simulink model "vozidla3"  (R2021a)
settings: Solver=VariableStepAuto  StartTime=0.0  StopTime=10  RelTol=1e-5
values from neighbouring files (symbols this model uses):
  Az = A-B*K    [appDekompLQR.m]    (also in appLQR.m; appSYM.m = A+B*K; appSZV.m = A+B*K; central_LQR.m)
  C = eye(pocet_stavu)    [appDekompLQR.m]    (also in appLQR.m; appSYM.m; appSZV.m; central_LQR.m)
  conds = [0 , 4 , 0 , 2 , 0, 1, 0, -1, 0]    [central_LQR.m]    (also in central_SYM.m = [0 , 4 , 0 , 3 , 0, 2, 0, -1, 0]; distri_STRUKTURAL.m = [0 , 4 , 0 , 3 , 0, 2, 0, -1, 0]; distri_SZV.m = [0 , 4 , 0 , 3 , 0, 2, 0, -1, 0]; porovnani_rizeni.m)
  conds0 = zeros(1,2*N-1)    [central_LQR.m]    (also in central_SYM.m; distri_STRUKTURAL.m = zeros(1,pocet_stavu); distri_SZV.m; porovnani_rizeni.m)
  D = zeros(pocet_stavu,N)    [appDekompLQR.m]    (also in appLQR.m; appSYM.m; appSZV.m; central_LQR.m)
  porucha = B    [appDekompLQR.m]    (also in appLQR.m; appSYM.m; appSZV.m; central_LQR.m)
libraries: simulink x1

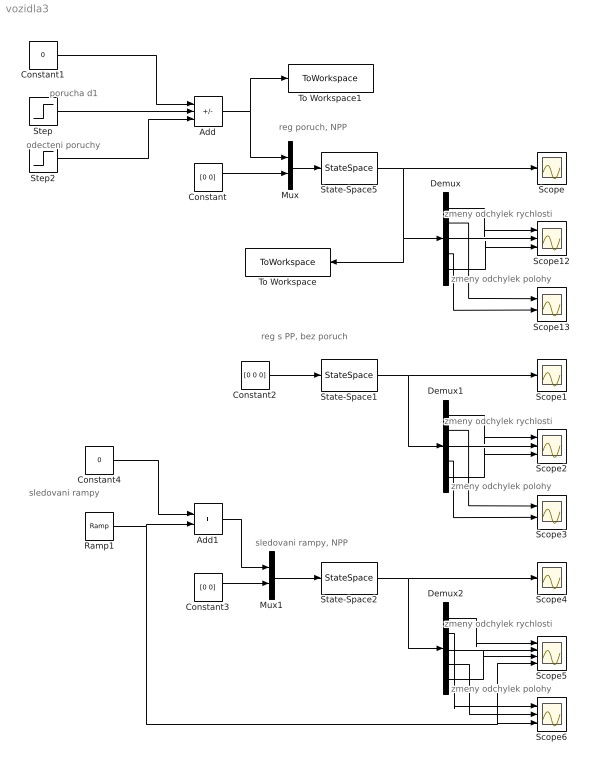
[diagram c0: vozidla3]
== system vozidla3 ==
  note: reg poruch, NPP
  note: reg s PP, bez poruch
  note: odecteni poruchy
  note: porucha d1
  note: zmeny odchylek polohy
  note: zmeny odchylek rychlosti
  note: zmeny odchylek polohy
  note: zmeny odchylek rychlosti
  note: sledovani rampy, NPP
  note: zmeny odchylek polohy
  note: zmeny odchylek rychlosti
  note: sledovani rampy
  Add : Sum  Inputs=++-
  Add1 : Sum
  Constant : Constant  Value=[0 0]
  Constant1 : Constant  Value=0
  Constant2 : Constant  Value=[0 0 0]
  Constant3 : Constant  Value=[0 0]
  Constant4 : Constant  Value=0
  Demux : Demux  Outputs=5
  Demux1 : Demux  Outputs=5
  Demux2 : Demux  Outputs=5
  Mux : Mux  Inputs=2
  Mux1 : Mux  Inputs=2
  Ramp1 : simulink/Sources/Ramp  slope=1  start=5  InitialOutput=0
  Scope : Scope
  Scope1 : Scope
  Scope12 : Scope  NumInputPorts=3
  Scope13 : Scope  NumInputPorts=2
  Scope2 : Scope  NumInputPorts=3
  Scope3 : Scope  NumInputPorts=2
  Scope4 : Scope
  Scope5 : Scope  NumInputPorts=4
  Scope6 : Scope  NumInputPorts=3
  State-Space1 : StateSpace  A=Az  B=porucha  C=C  D=D  InitialCondition=conds
  State-Space2 : StateSpace  A=Az  B=porucha  C=C  D=D  InitialCondition=conds0
  State-Space5 : StateSpace  A=Az  B=porucha  C=C  D=D  InitialCondition=conds0
  Step : Step  Time=5  After=2  SampleTime=0
  Step2 : Step  Time=6  After=2  SampleTime=0
  To Workspace : ToWorkspace  VariableName=stavy  SaveFormat=Structure  SampleTime=-1
  To Workspace1 : ToWorkspace  VariableName=vstup  SaveFormat=Structure  SampleTime=-1
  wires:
  State-Space5/1 -> Scope/1, To Workspace/1, Demux/1
  Demux/1 -> Scope12/1
  Demux/3 -> Scope12/2
  Demux/5 -> Scope12/3
  Demux/2 -> Scope13/1
  Demux/4 -> Scope13/2
  Step/1 -> Add/2
  Mux/1 -> State-Space5/1
  Step2/1 -> Add/3
  Constant1/1 -> Add/1
  Constant/1 -> Mux/2
  State-Space1/1 -> Demux1/1, Scope1/1
  Demux1/5 -> Scope2/3
  Demux1/4 -> Scope3/2
  Demux1/1 -> Scope2/1
  Demux1/3 -> Scope2/2
  Demux1/2 -> Scope3/1
  Constant2/1 -> State-Space1/1
  Add/1 -> To Workspace1/1, Mux/1
  Constant3/1 -> Mux1/2
  Constant4/1 -> Add1/1
  Mux1/1 -> State-Space2/1
  State-Space2/1 -> Demux2/1, Scope4/1
  Demux2/5 -> Scope5/3
  Demux2/4 -> Scope6/2
  Demux2/1 -> Scope5/1
  Demux2/3 -> Scope5/2
  Demux2/2 -> Scope6/1
  Ramp1/1 -> Scope5/4, Scope6/3, Add1/2
  Add1/1 -> Mux1/1
